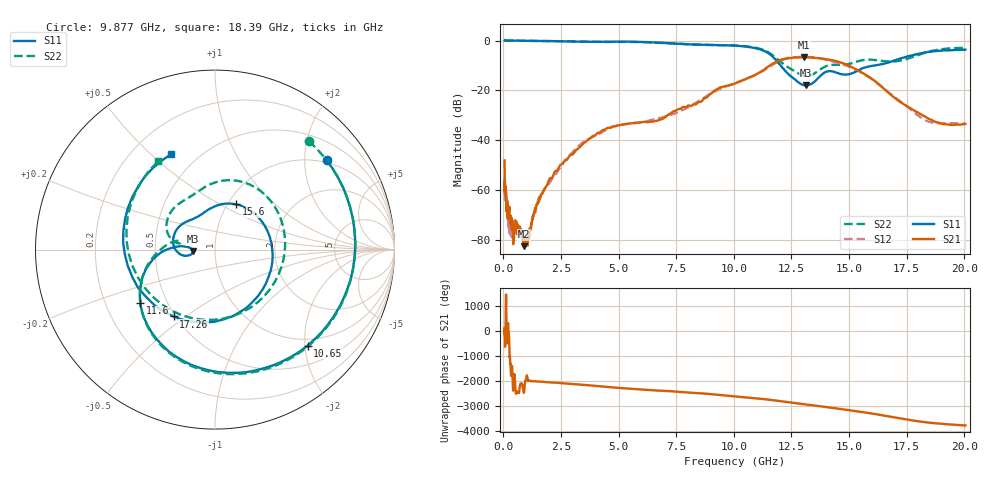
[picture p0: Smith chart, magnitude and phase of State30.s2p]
# Hz S DB R 50
!freq MagS11 AngS11 MagS21 AngS21 MagS12 AngS12 MagS22 AngS22
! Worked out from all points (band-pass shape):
!   1601 points, 50 MHz to 20.05 GHz, reference 50 ohm
!   highest |S21| = -6.68 dB at 13.03 GHz (marker M1); lowest = -82.6 dB at 904.9 MHz (marker M2)
!   |S21| within 3 dB of the highest: 11.62 GHz to 14.89 GHz (3.266 GHz wide, 24.6 % of centre)
!   lowest |S11| = -18.1 dB at 13.13 GHz (marker M3), VSWR 1.29, Z = 38.9 - j0.694 ohm
!   |S11| at or under -10 dB: 12.02 GHz to 16.13 GHz (4.109 GHz wide, 29.2 % of centre)
!   |S22| runs from -14.2 to 0.0 dB; largest |S21 - S12| = 0.025
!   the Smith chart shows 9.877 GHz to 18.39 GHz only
!   S11 on the Smith chart (normalised r, x): 9.877 GHz: 0.93, +2.54; 10.65 GHz: 0.86, -2.05; 11.6 GHz: 0.35, -0.29; 15.6 GHz: 1.09, +0.60; 17.26 GHz: 0.49, -0.45; 18.39 GHz: 0.36, +0.58
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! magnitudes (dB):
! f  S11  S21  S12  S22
! 50 MHz  0.0  -48.2  -64.2  0.0
! 53.09 MHz  0.0  -54.9  -54.9  0.0
! 59.85 MHz  0.0  -60.5  -58.1  0.0
! 105.8 MHz  0.0  -59.7  -60.8  0.0
! 135.9 MHz  0.0  -67.1  -66.1  0.0
! 251.3 MHz  0.0  -67.7  -70.4  0.0
! 369.6 MHz  0.0  -75.7  -78.8  0.0
! 429.4 MHz  0.0  -81.1  -75.0  0.0
! 510.1 MHz  0.0  -75.3  -73.6  -0.1
! 904.9 MHz  -0.1  -82.6  -78.6  -0.1
! 1.005 GHz  -0.1  -81.1  -80.3  -0.1
! 2.722 GHz  -0.3  -48.0  -47.8  -0.4
! 7.402 GHz  -1.2  -28.4  -29.4  -1.2
! 9.877 GHz  -2.0  -17.8  -17.7  -1.9
! 10.65 GHz  -2.6  -15.0  -15.0  -2.5
! 11.6 GHz  -5.8  -9.8  -10.3  -5.4
! 13.03 GHz  -18.0  -6.7  -6.6  -14.1
! 13.13 GHz  -18.1  -6.8  -6.6  -14.2
! 15.6 GHz  -11.1  -13.1  -13.3  -7.9
! 17.26 GHz  -7.2  -24.9  -24.6  -8.0
! 18.39 GHz  -4.7  -31.1  -32.4  -4.6
! 20.05 GHz  -3.7  -33.5  -33.4  -2.9
